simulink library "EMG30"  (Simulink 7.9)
settings: Solver=ode45  StartTime=0.0  StopTime=10.0  RelTol=1e-3

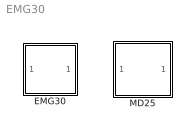
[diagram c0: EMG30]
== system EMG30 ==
  EMG30 : Subsystem  mask(Permanent Magnet Electric Motor Model - EMG30){R=7.101, L=0.0034, J=0.0019, b=0.000931, Kt=0.509, Ke=0.509, Tc=0.04}
      mask prompts: R "Resistance (R)"; L "Indutance (L)"; J "Inertia Moment (J)"; b "Viscous Friction (b)"; Kt "Torque Contant (Kt)"; Ke "Back E.M.F. Contant (Ke)"; Tc "Viscous Torque"
      mask help: Mathematical model for the EMG30 permanent magnet electric motor. Currently this is a very popular motor for robotic applications. (c)2013 João Paulo Coelho wwww.ipb.pt/~jpcoelho
  MD25 : Subsystem  mask{A=60}
      mask prompts: A "Acceleration"

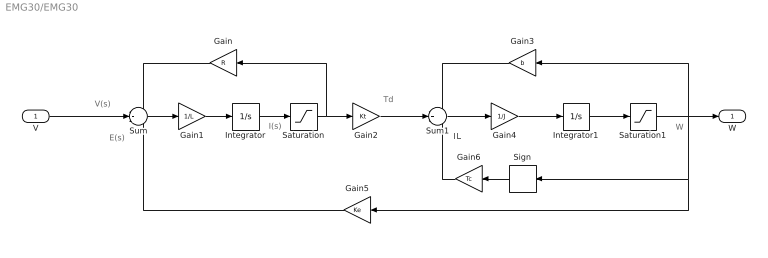
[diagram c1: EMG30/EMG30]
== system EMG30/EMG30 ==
  note: V(s)
  note: E(s)
  note: I(s)
  note: Td
  note: TL
  note: W
  V : Inport
  Gain : Gain  Gain=R
  Gain1 : Gain  Gain=1/L
  Gain2 : Gain  Gain=Kt
  Gain3 : Gain  Gain=b
  Gain4 : Gain  Gain=1/J
  Gain5 : Gain  Gain=Ke
  Gain6 : Gain  Gain=Tc
  Integrator : Integrator
  Integrator1 : Integrator
  Saturation : Saturate  UpperLimit=1.7  LowerLimit=-1.7  ZeroCross=off
  Saturation1 : Saturate  UpperLimit=22  LowerLimit=-22  ZeroCross=off
  Sign : Signum  ZeroCross=off
  Sum : Sum  Inputs=-+-
  Sum1 : Sum  Inputs=-+-
  W : Outport
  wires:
  V/1 -> Sum/2
  Gain/1 -> Sum/1
  Sum/1 -> Gain1/1
  Gain1/1 -> Integrator/1
  Gain2/1 -> Sum1/2
  Gain3/1 -> Sum1/1
  Sum1/1 -> Gain4/1
  Gain4/1 -> Integrator1/1
  Gain5/1 -> Sum/3
  Sign/1 -> Gain6/1
  Gain6/1 -> Sum1/3
  Integrator1/1 -> Saturation1/1
  Integrator/1 -> Saturation/1
  Saturation/1 -> Gain2/1, Gain/1
  Saturation1/1 -> W/1, Gain3/1, Sign/1, Gain5/1

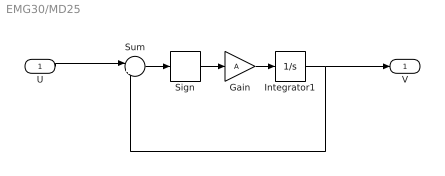
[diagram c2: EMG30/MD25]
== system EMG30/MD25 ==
  U : Inport
  Gain : Gain  Gain=A
  Integrator1 : Integrator
  Sign : Signum  ZeroCross=off
  Sum : Sum  Inputs=|+-
  V : Outport
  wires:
  Sum/1 -> Sign/1
  Integrator1/1 -> Sum/2, V/1
  Sign/1 -> Gain/1
  Gain/1 -> Integrator1/1
  U/1 -> Sum/1
